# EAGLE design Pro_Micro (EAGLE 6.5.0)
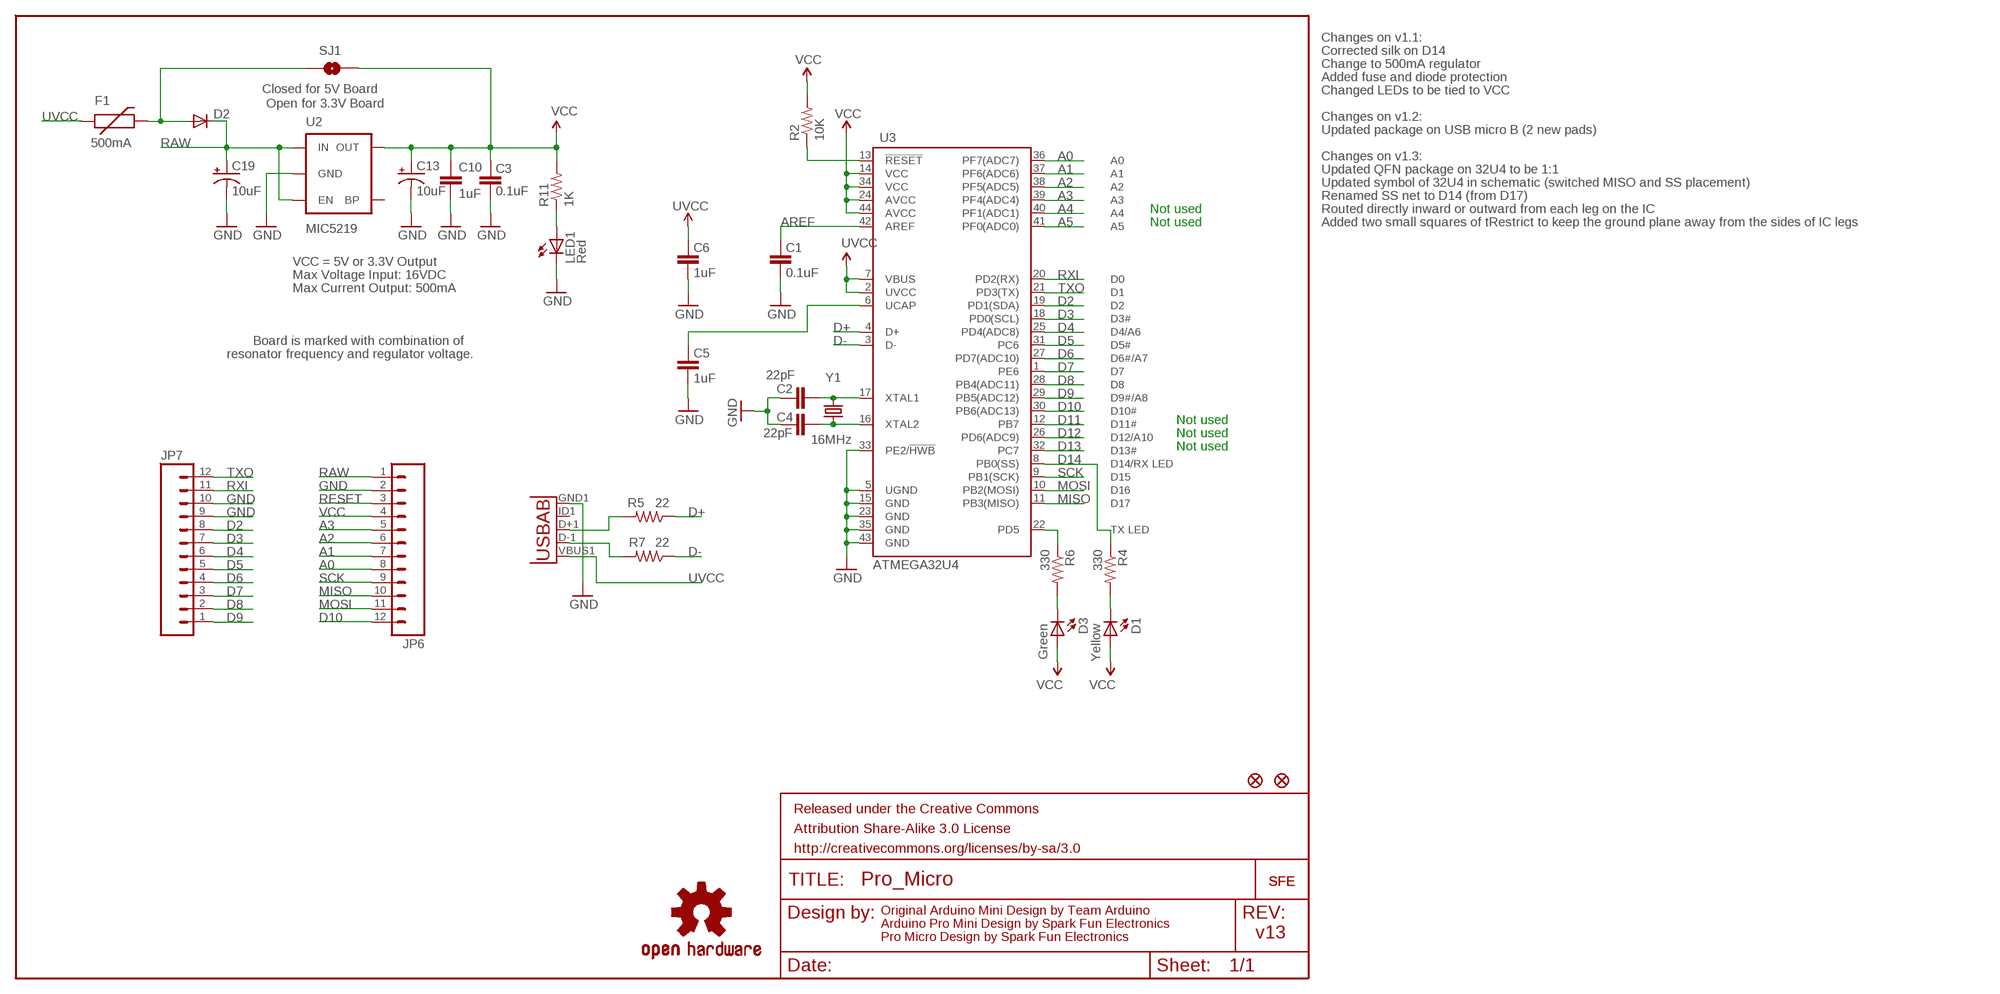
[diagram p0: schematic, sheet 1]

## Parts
C1  0.1uF  CAP0603-CAP  [0603-CAP]
C2  22pF  CAP0603-CAP  [0603-CAP]
C3  0.1uF  CAP0603-CAP  [0603-CAP]
C4  22pF  CAP0603-CAP  [0603-CAP]
C5  1uF  CAP0603-CAP  [0603-CAP]
C6  1uF  CAP0603-CAP  [0603-CAP]
C10  1uF  CAP0603-CAP  [0603-CAP]
C13  10uF  CAP_POL1206  [EIA3216]
C19  10uF  CAP_POL1206  [EIA3216]
D1  Yellow  LED0603  [LED-0603]
D2  DIODESOD  [SOD-323]
D3  Green  LED0603  [LED-0603]
F1  500mA  PTCSMD  [PTC-1206]
FRAME1  FRAME-LETTER  [CREATIVE_COMMONS]
JP1  FIDUCIALUFIDUCIAL  [MICRO-FIDUCIAL]
JP2  FIDUCIALUFIDUCIAL  [MICRO-FIDUCIAL]
JP6  M12PTH  [1X12]
JP7  M12PTH  [1X12]
LED1  Red  LED0603  [LED-0603]
R2  10K  RESISTOR0603-RES  [0603-RES]
R4  330  RESISTOR0603-RES  [0603-RES]
R5  22  RESISTOR0603-RES  [0603-RES]
R6  330  RESISTOR0603-RES  [0603-RES]
R7  22  RESISTOR0603-RES  [0603-RES]
R11  1K  RESISTOR0603-RES  [0603-RES]
SJ1  Closed for 5V Board  SOLDERJUMPERNO  [SJ_2S-NO]
U2  MIC5219  V_REG_LDOSMD  [SOT23-5]
U3  ATMEGA32U4  ATMEGA32U4OUTFAKES  [QFN-44-NOPAD_1:1-OUTFAKES]
U$1  LOGO-SFESK  [SFE-LOGO-FLAME]
U$3  OSHW-LOGOS  [OSHW-LOGO-S]
U$11  LOGO-SFENEW  [SFE-NEW-WEBLOGO]
X1  USB-ABIN&OUT  [USB-AB-MICRO-SMD-V03-IN&OUT]
Y1  16MHz  CRYSTAL5X3  [CRYSTAL-SMD-5X3]

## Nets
A0: JP6.8 U3.36(PF7(ADC7))
A1: JP6.7 U3.37(PF6(ADC6))
A2: JP6.6 U3.38(PF5(ADC5))
A3: JP6.5 U3.39(PF4(ADC4))
A4: U3.40(PF1(ADC1))
A5: U3.41(PF0(ADC0))
AREF: C1.2 U3.42(AREF)
D2: JP7.8 U3.19(PD1(SDA))
D3: JP7.7 U3.18(PD0(SCL))
D4: JP7.6 U3.25(PD4(ADC8))
D5: JP7.5 U3.31(PC6)
D6: JP7.4 U3.27(PD7(ADC10))
D7: JP7.3 U3.1(PE6)
D8: JP7.2 U3.28(PB4(ADC11))
D9: JP7.1 U3.29(PB5(ADC12))
D10: JP6.12 U3.30(PB6(ADC13))
D11: U3.12(PB7)
D12: U3.26(PD6(ADC9))
D13: U3.32(PC7)
D14: R4.1 U3.8(PB0(SS))
D+: R5.1 U3.4(D+)
D-: R7.1 U3.3(D-)
GND [vcc]: C1.1 C2.2 C3.1 C4.2 C5.1 C6.1 C10.2 C13.C(-) C19.C(-) JP6.2 JP7.9 JP7.10 LED1.C U2.2(GND) U3.5(UGND) U3.15(GND) U3.23(GND) U3.33(PE2/!HWB) U3.35(GND) U3.43(GND) X1.GND1(GND)
MISO: JP6.10 U3.11(PB3(MISO))
MOSI: JP6.11 U3.10(PB2(MOSI))
N$1: C4.1 U3.16(XTAL2) Y1.1
N$2: C2.1 U3.17(XTAL1) Y1.3
N$3: D2.2(A) F1.2 SJ1.1
N$4: C5.2 U3.6(UCAP)
N$5: D1.C R4.2
N$6: R7.2 X1.D-1(D-)
N$7: D3.C R6.2
N$8: R5.2 X1.D+1(D+)
N$38: LED1.A R11.1
RAW [vcc]: C19.A(+) D2.1(C) JP6.1 U2.1(IN) U2.3(EN)
RESET: JP6.3 R2.1 U3.13(!RESET)
RXI: JP7.11 U3.20(PD2(RX))
SCK: JP6.9 U3.9(PB1(SCK))
TXLED: R6.1 U3.22(PD5)
TXO: JP7.12 U3.21(PD3(TX))
UVCC: C6.2 F1.1 U3.2(UVCC) U3.7(VBUS) X1.VBUS1(VBUS)
VCC: C3.2 C10.1 C13.A(+) D1.A D3.A JP6.4 R2.2 R11.2 SJ1.2 U2.5(OUT) U3.14(VCC) U3.24(AVCC) U3.34(VCC) U3.44(AVCC)
Unconnected: U2.4(BP) X1.ID1(USBID)

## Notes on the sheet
- Changes on v1.1:
- Corrected silk on D14
- Change to 500mA regulator
- Added fuse and diode protection
- Changed LEDs to be tied to VCC
- Open for 3.3V Board
- Changes on v1.2:
- Updated package on USB micro B (2 new pads)
- Changes on v1.3:
- Updated QFN package on 32U4 to be 1:1
- Updated symbol of 32U4 in schematic (switched MISO and SS placement)
- Renamed SS net to D14 (from D17)
- Not used | Routed directly inward or outward from each leg on the IC
- Not used | Added two small squares of tRestrict to keep the ground plane away from the sides of IC legs
- VCC = 5V or 3.3V Output
- Max Voltage Input: 16VDC
- Max Current Output: 500mA
- Board is marked with combination of
- resonator frequency and regulator voltage.
- Not used
- Not used
- Not used
- Original Arduino Mini Design by Team Arduino
- Arduino Pro Mini Design by Spark Fun Electronics
- Pro Micro Design by Spark Fun Electronics | v13

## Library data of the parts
C1-C6 C10 = SparkFun:CAP: Capacitor
C13 C19 = SparkFun:CAP_POL: Capacitor Polarized
D1 D3 LED1 = SparkFun:LED: LEDs
D2 = SparkFun:DIODE: Diode
F1 = SparkFun:PTC: Resettable Fuse PTC
FRAME1 = SparkFun-Aesthetics:FRAME-LETTER: Schematic Frame
JP1 JP2 = SparkFun:FIDUCIAL: Fiducial Alignment Points
JP6 JP7 = SparkFun:M12: Header 12 Standard 12-pin 0.1" header. Use with straight break away headers (SKU : PRT-00116), right angle break away headers (PRT-00553), swiss pins (PRT-00743), machine pins (PRT-00117), and female headers (PRT-00115).
R2 R4-R7 R11 = SparkFun:RESISTOR: Resistor
SJ1 = SparkFun:SOLDERJUMPER: Solder Jumper
U2 = SparkFun:V_REG_LDO: Voltage Regulator LDO Standard 150mA LDO voltage regulator in SOT-23 layout. Micrel part MIC5205. BP (by-pass) pin is used to lower output noise with 470pF cap.
U3 = Testing:ATMEGA32U4: Atmel 44-pin 8-bit Microcontroller with 32KBytes of ISP Flash and USB Controller
U$1 U$11 = SparkFun:LOGO-SFE: Spark Fun Electronics PCB Logo
U$3 = SparkFun:OSHW-LOGO: Open Source Hardware Logo This logo indicates the piece of hardware it is found on incorporates a OSHW license and/or adheres to the definition of open source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
X1 = Testing:USB-AB: This is a USB AB connector that is compatible with USB OTG. i.e. this connector can serve as a host or device
Y1 = SparkFun:CRYSTAL: Crystals

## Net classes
0 default: width 0.203 mm

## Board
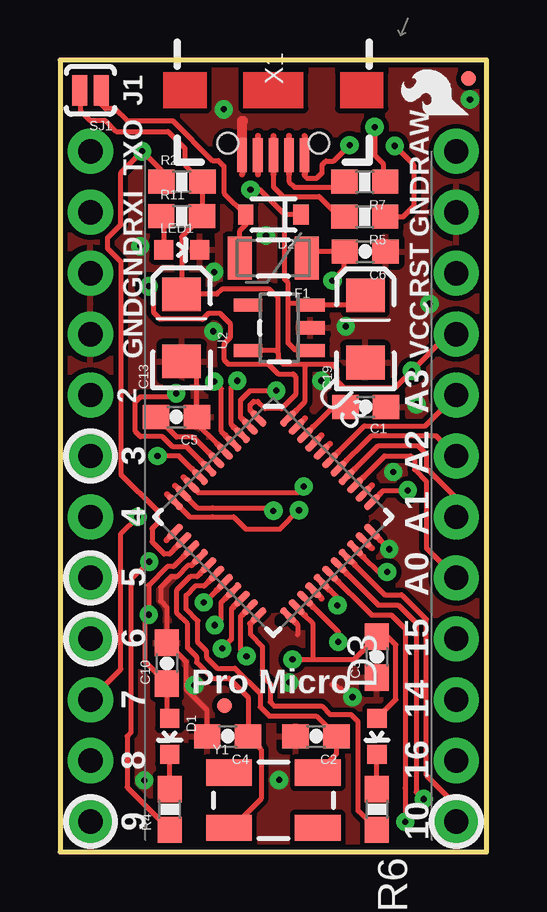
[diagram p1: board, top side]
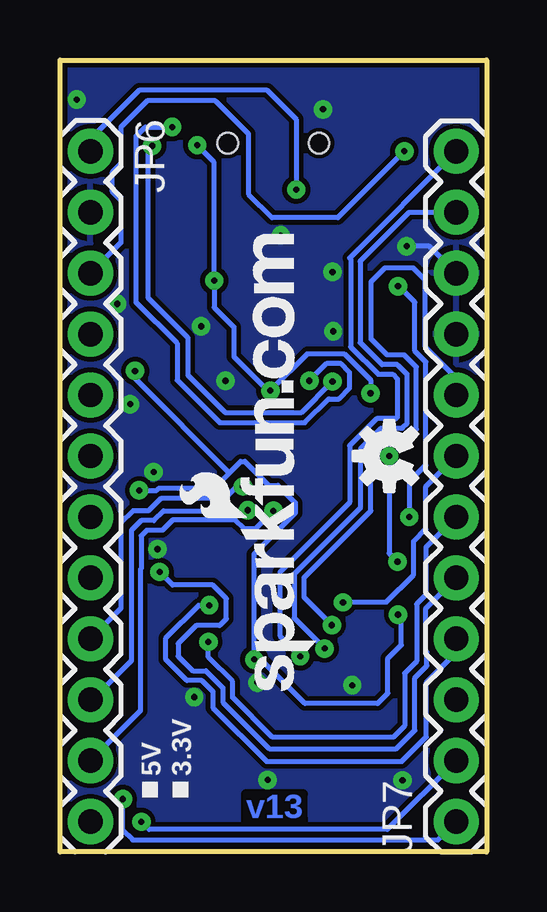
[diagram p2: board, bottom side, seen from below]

Size 17.78 x 33.02 mm. Coordinates in mm from the lower left corner, seen from the top.
Outline: 0,33.02 0,0 17.78,0 17.78,33.02 0,33.02
Copper layers (1*16): Top 0.035mm / dielectric 1.5mm / Bottom 0.035mm
Design rules "SparkFun *": minimum track width 8mil, minimum drill 15mil, track to track 7mil, track to pad 7mil, pad to pad 7mil, via to via 7mil, smd to smd 7mil, copper to edge 7mil, drill to drill 7mil, minimum pad ring 12mil, minimum via ring 10mil, stop-mask expansion 4mil, vias tented up to drill 20mil, thermal gap 10mil
tRestrict: area 9.1,9.6 to 9.3,9.7; area 13.1,13.6 to 13.1,13.7; area 5.5,10.3 to 12.6,17.6

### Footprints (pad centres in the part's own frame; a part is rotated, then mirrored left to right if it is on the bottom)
0603-CAP = smd 1.1 x 1: 1 -0.85,0; 2 0.85,0
EIA3216 = smd 1.4 x 1.6: A 1.4,0; C -1.4,0
LED-0603 = smd 0.8 x 0.8: A 0,-0.75; C 0,0.75
SOD-323 = smd 0.63 x 0.83: 1 -1.15,0; 2 1.15,0
PTC-1206 = smd 1 x 1.8: 1 -1.4,0; 2 1.4,0
MICRO-FIDUCIAL = smd 0.635 x 0.635: 1 0,0
1X12 = drill 1.016 pad 1.88: 1 0,0; 2 2.54,0; 3 5.08,0; 4 7.62,0; 5 10.16,0; 6 12.7,0; 7 15.24,0; 8 17.78,0; 9 20.32,0; 10 22.86,0; 11 25.4,0; 12 27.94,0
0603-RES = smd 1.1 x 1: 1 -0.85,0; 2 0.85,0
SJ_2S-NO = smd 0.635 x 1.27: 1 -0.45,0; 2 0.45,0
SOT23-5 = smd 0.55 x 1.2: 1 -0.95,-1.3; 2 0,-1.3; 3 0.95,-1.3; 4 0.95,1.3; 5 -0.95,1.3
QFN-44-NOPAD_1:1-OUTFAKES = smd 0.8 x 0.3: 1 -3.337,2.465; 2 -3.337,1.972; 3 -3.337,1.479; 4 -3.337,0.986; 5 -3.337,0.493; 6 -3.337,0; 7 -3.337,-0.493; 8 -3.337,-0.986; 9 -3.337,-1.479; 10 -3.337,-1.972; 11 -3.337,-2.465; 23 3.337,-2.465; 24 3.337,-1.972; 25 3.337,-1.479; 26 3.337,-0.986; 27 3.337,-0.493; 28 3.337,0; 29 3.337,0.493; 30 3.337,0.986; 31 3.337,1.479; 32 3.337,1.972; 33 3.337,2.465 | smd 0.3 x 0.8: 12 -2.465,-3.337; 13 -1.972,-3.337; 14 -1.479,-3.337; 15 -0.986,-3.337; 16 -0.493,-3.337; 17 0,-3.337; 18 0.493,-3.337; 19 0.986,-3.337; 20 1.479,-3.337; 21 1.972,-3.337; 22 2.465,-3.337; 34 2.465,3.337; 35 1.972,3.337; 36 1.479,3.337; 37 0.986,3.337; 38 0.493,3.337; 39 0,3.337; 40 -0.493,3.337; 41 -0.986,3.337; 42 -1.479,3.337; 43 -1.972,3.337; 44 -2.465,3.337
USB-AB-MICRO-SMD-V03-IN&OUT = smd 1.4 x 0.4: D+1 2.7,0; D-1 2.7,0.65; GND1 2.7,-1.3; ID1 2.7,-0.65; VBUS1 2.7,1.3 | hole 0.85: 2.2,1.9; 2.2,-1.9
CRYSTAL-SMD-5X3 = smd 1.9 x 1.1: 1 -1.85,-1.15; 2 1.85,-1.15; 3 1.85,1.15; 4 -1.85,1.15

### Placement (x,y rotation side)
C1  12.74,18.56 180 top
C2  10.67,4.83 180 top
C3  13.21,8.13 90 top
C4  6.99,4.83 180 top
C5  4.85,18.14 180 top
C6  12.71,25.03 180 top
C10  4.46,7.87 90 top
C13  5.07,21.85 90 top
C19  12.72,21.8 90 top
D1  4.57,4.83 180 top
D2  8.89,26.57 180 top
D3  13.21,4.83 180 top
F1  8.89,24.77 180 top
FRAME1  not placed on the board
JP1  6.86,6.1 0 top
JP2  17.02,32.26 0 top
JP6  16.51,29.21 270 bottom
JP7  1.27,1.27 90 bottom
LED1  5.07,25.11 270 top
R2  5.08,27.94 0 top
R4  4.57,1.78 90 top
R5  12.7,26.49 180 top
R6  13.21,1.78 90 top
R7  12.7,27.94 180 top
R11  5.07,26.5 0 top
SJ1  1.27,31.75 180 top
U2  9.14,21.85 90 top
U3  8.89,13.97 315 top
U$1  17.02,30.73 90 top
U$3  4.06,16.51 90 bottom
U$11  7.11,6.73 90 bottom
X1  8.89,31.75 270 top
Y1  8.89,2.16 0 top

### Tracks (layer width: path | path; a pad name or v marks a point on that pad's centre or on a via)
A0
  Top 0.203: U3.36 13.53,16.52 14.61,16.52 14.78,16.35 14.78,15.94 15.27,15.45 15.27,12.67 JP6.8
A1
  Top 0.203: U3.37 13.26,16.95 14.91,16.95 15.27,16.59 15.27,16.01 16.51,14.77 JP6.7
A2
  Top 0.203: U3.38 12.98,17.36 15.66,17.36 JP6.6
A3
  Top 0.203: 12.68,17.77 12.69,17.77 | 11.6,16.68 12.69,17.77 | 12.69,17.77 15.22,17.77 JP6.5
AREF
  Top 0.203: 10.55,17.72 11.39,18.56 C1.2
D2  (via drill 0.25)
  Top 0.203: 6.88,10.56 6.71,10.39 6.71,9.72 v6.45,9.46
  Bottom 0.203: v6.45,9.46 7.62,10.63 7.62,11.43 4.83,14.22 4.83,16.69 4.23,17.29 3.28,17.29 2.93,17.63 2.93,20.22 3.44,20.73 4.15,20.73 4.82,21.4 4.82,23.77 4.83,23.77 4.25,24.35 3.06,24.35 2.55,23.85 2.55,21.05 1.27,19.76 JP7.8
D3  (via drill 0.25)
  Top 0.203: 6.53,10.91 6.02,10.41 v5.99,10.41
  Bottom 0.203: JP7.7 2.54,15.24 2.54,13.46 3.05,12.95 3.05,11.56 4.2,10.41 v5.99,10.41
D4  (via drill 0.25)
  Top 0.203: 10.55,10.22 11.6,9.17 v11.6,8.76
  Bottom 0.203: JP7.6 2.54,12.7 2.54,10.72 2.92,10.34 2.92,7.95 3.42,7.45 3.42,5.26 3.89,4.79 8.93,4.79 10.58,6.45 10.58,7.1 11.6,8.12 v11.6,8.76
D5  (via drill 0.25)
  Top 0.203: 12.64,12.31 13.28,11.68 v13.63,11.68
  Bottom 0.203: JP7.5 2.54,10.16 2.54,8.38 2.5,8.34 2.5,7.76 3,7.27 3,5.07 3.76,4.3 9.05,4.3 11,6.25 11,6.86 11.01,6.86 11.71,7.55 12.25,7.55 12.86,8.16 12.86,8.69 12.11,9.44 11.13,9.44 10.85,9.73 10.85,10.57 11.41,11.13 13.09,11.13 v13.63,11.68
D6  (via drill 0.25)
  Top 0.203: v11.56,10.29 11.56,10.6 v11.56,10.29 | U3.27 11.56,10.61 v11.56,10.29
  Bottom 0.203: v11.56,10.29 12.01,10.29 13.37,8.92 13.37,8.03 12.49,7.15 11.87,7.15 11.41,6.69 11.41,6.02 9.17,3.78 3.53,3.78 2.51,4.8 2.51,7.07 1.27,8.31 JP7.4
D7  (via drill 0.25)
  Top 0.203: JP7.3 2.54,7.62 2.54,13.28 v3.23,13.97 | v3.7,23.59 3.7,23.54 3.91,23.32 3.91,22.48 4.17,22.22 5.95,22.22 6.19,22.46 6.66,22.46 7.09,22.04 7.09,21.44 6.84,21.2 6.84,20.51 7.03,20.33 8.71,20.33 8.71,20.31 9.1,19.93 9.72,19.93 9.82,19.83 9.82,19.07 9.24,18.49 8.54,18.49 8.24,18.79 8.07,18.79 7.92,18.64 7.92,18.43 U3.1 7.93,18.42
  Bottom 0.203: v3.7,23.59 3.67,23.59 3,22.92 3,20.89 2.54,20.43 2.54,16.13 3.23,15.44 v3.23,13.97
D8  (via drill 0.25)
  Top 0.203: U3.28 12.98,9.88 13.8,9.88 14.38,9.31 14.38,2.67 14.39,2.65 v14.39,1.26
  Bottom 0.203: JP7.2 4.14,0.94 14.07,0.94 v14.39,1.26
D9  (via drill 0.25)
  Top 0.203: 11.95,11.61 13.26,10.3 14.08,10.3 14.83,9.55 14.83,2.49 15.12,2.21 v15.16,2.21
  Bottom 0.203: JP7.1 2.03,0.51 14.76,0.51 15.16,0.91 v15.16,2.21
D10
  Top 0.203: JP6.12 16.51,1.96 15.27,3.2 15.27,9.7 14.24,10.73 13.53,10.73 U3.30
D14  (via drill 0.25)
  Top 0.203: R4.1 2.79,2.71 2.79,4.83 2.95,4.98 2.95,11.34 v3.72,12.1 | 5.5,15.97 4.96,16.51 v4.06,16.51
  Bottom 0.203: v4.06,16.51 4.06,12.45 v3.72,12.1
D+  (via drill 0.25)
  Top 0.203: v13.95,29.44 14.73,28.65 14.73,26.92 14.29,26.49 R5.1 | U3.4 6.72,17.53 6.72,19.32 v6.43,19.61
  Bottom 0.203: v13.95,29.44 14.1,29.29 14.1,23.09 12.45,21.44 12.45,19.88 10.91,18.34 10.91,18.32 7.72,18.32 v6.43,19.61
D-  (via drill 0.25)
  Top 0.203: 13.55,28.26 R7.1 13.46,28.03 13.46,28.7 13.11,29.06 v13.11,30.23 | v7.39,19.65 7.14,19.39 7.14,17.81 7.24,17.71
  Bottom 0.203: v13.11,30.23 14.22,30.23 14.61,29.84 14.61,22.91 12.9,21.21 12.9,19.67 11.12,17.9 7.57,17.9 6.58,18.89 6.18,18.89 6.17,18.88 5.72,19.34 5.72,20 6.07,20.36 6.68,20.36 v7.39,19.65
GND  (via drill 0.25)
  Top 0.203: v13.71,12.62 v13.72,12.62 | U3.33 13.65,12.7 13.97,12.7 | C3.1 13.21,7.47 | 5.49,11.96 5.36,11.96 4.9,11.5 4.66,11.5 4.2,11.03 4.2,10.46 4.46,10.2 C10.2 4.63,8.55 4.64,8.55 5.26,7.92 5.26,6.78 6.13,5.91 C4.2 | 9.86,9.52 9.91,9.47 9.91,9.07 | 11.34,6.98 arc-21 v12.19,6.46 | 5.38,20.45 C13.C 5.7,19.82 C5.1 5.7,17.85 6.54,17.02
  Top 0.406: X1.GND1 7.59,30.48 7.62,30.48
  Bottom 0.203: JP7.10 2.39,25.25 v3.34,25.25
  other vias: 9.13,3 14.86,18.67 11.9,21.92 13.88,15.84 10.88,19.65 6.39,21.71 17.08,31.37 8.58,25.7 15.4,22.85 6.82,30.96 3.51,2.99 5.6,6.95 6.43,24.18 9.56,7.06
  pour Top (isolate 0.203): 0,33.02 17.78,33.02 17.78,0 0,0
  pour Bottom (isolate 0.203): 0,33.02 17.78,33.02 17.78,0 0,0
MISO  (via drill 0.25)
  Top 0.203: v9.96,14.25 9.17,13.46 7.75,13.46 7.24,13.97 6.35,13.97 5.42,13.97 5.4,13.97 U3.11
  Bottom 0.203: JP6.10 16.43,6.35 14.81,7.98 14.81,13.41 14.4,13.82 13.87,13.82 13.46,14.22 9.98,14.22 v9.96,14.25
MOSI  (via drill 0.25)
  Top 0.203: v8.89,14.22 8.76,14.35 6.35,14.35 5.74,14.35 5.72,14.35 U3.10
  Bottom 0.203: JP6.11 14.43,5.89 14.43,11.79 14.4,11.81 14.4,13.18 14.17,13.41 13.51,13.41 13.08,13.84 10.49,13.84 10.11,13.46 9.65,13.46 v8.89,14.22
N$1
  Top 0.203: Y1.1 7.17,1.01 8.38,2.22 8.38,4.28 C4.1 7.83,6.45 7.05,7.24 6.35,7.24 5.69,7.9 5.69,8.14 5.32,8.51 5.32,9.51 4.85,9.98 4.85,10.9 | 5.83,11.61 5.71,11.49 5.44,11.49 4.85,10.9 | 4.85,10.9
N$2
  Top 0.203: Y1.3 11.52,4.09 C2.1 10.68,5.67 8.71,5.67 8.34,6.04 8.34,6.61 7.29,7.67 6.55,7.67 6.1,8.12 6.1,8.37 5.74,8.73 5.74,9.64 5.25,10.13 5.25,10.71 5.63,11.09 6,11.09 6.18,11.26
N$3
  Top 0.203: F1.2 7.49,25.91 7.74,26.16 D2.2 6.83,27.48 6.83,28.6 6.6,28.83 6.35,28.83 4.7,30.48 2.79,30.48 2.29,30.99 1.91,30.99 1.68,31.21 SJ1.1
N$4
  Top 0.203: C5.2 4.03,18.14 4.86,17.3 5.56,17.3 U3.6
N$5
  Top 0.203: R4.2 D1.C
N$6
  Top 0.203: X1.D-1 9.54,27.95 9.78,27.71 11.65,27.71 11.85,27.91 R7.2
N$7
  Top 0.203: R6.2 D3.C
N$8
  Top 0.203: X1.D+1 8.89,27.74 9.3,27.33 10.79,27.33 11.64,26.49 R5.2
N$38
  Top 0.203: R11.1 4.32,26.4 LED1.A
RAW  (via drill 0.25)
  Top 0.203: 9.51,22.86 9.51,21.21 9.78,20.94 10.4,20.94 U2.1 | D2.1 9.37,26.57 | 9.37,26.57 8.33,27.61 v7.94,27.61 | C19.A 12.32,22.8 U2.3 10.38,22.86 9.51,22.86 | 9.51,22.86 9.51,23.73 9.36,23.88 9.36,26.56 9.37,26.57
  Bottom 0.203: JP6.1 16.51,29.72 14.48,31.75 9.14,31.75 7.94,30.54 v7.94,27.61
RESET  (via drill 0.25)
  Top 0.203: 4.79,12.66 4.71,12.58 4.71,12.57 4.56,12.42 4.34,12.42 3.83,12.93 3.83,13.49 4.06,13.72 4.06,14.22 2.54,15.75 2.54,24.61 1.98,25.17 1.98,25.59 2.54,26.15 2.54,28.32 v3.43,29.21 4.23,28.41 R2.1
  Bottom 0.203: JP6.3 15.24,25.4 15.24,27.18 15.62,27.56 15.62,28.32 15.24,28.7 15.24,30.23 14.15,31.32 11.3,31.32 9.93,29.95 9.93,27.43 8.94,26.44 6.2,26.44 v3.43,29.21
RXI  (via drill 0.25)
  Top 0.203: 7.23,10.22 7.14,10.13 7.14,8.87 v6.75,8.48
  Bottom 0.203: JP7.11 3.23,26.67 5.27,24.63 5.27,21.23 4.36,20.32 3.72,20.32 3.72,20.31 3.32,19.91 3.32,17.87 3.52,17.67 | v6.75,8.48 8.03,9.76 8.03,11.6 5.26,14.37 5.26,16.82 4.4,17.67 3.52,17.67 | 3.52,17.67 3.51,17.67
SCK  (via drill 0.25)
  Top 0.203: v10.16,15.24 9.91,14.99 6.35,14.99 5.78,14.99 | 5.75,14.99 5.78,14.99 | U3.9 5.78,14.99
  Bottom 0.203: JP6.9 15.24,10.16 15.24,13.72 14.73,14.22 14.1,14.22 13.59,14.73 10.92,14.73 10.41,15.24 v10.16,15.24
TXLED
  Top 0.203: 7.92,9.52 7.93,9.53 7.94,9.53 7.94,9.05 8.44,8.55 8.44,7.34 8.75,7.03 8.75,6.25 8.91,6.09 10.9,6.09 11.27,5.72 12.13,5.72 12.42,5.44 12.42,1.72 R6.1
TXO  (via drill 0.25)
  Top 0.203: 7.58,9.87 7.54,9.83 7.52,9.83 7.52,8.41 v7.77,8.16
  Bottom 0.203: JP7.12 5.71,24.77 5.67,24.72 5.67,21.05 4.53,19.92 3.92,19.92 3.72,19.72 3.72,18.13 3.79,18.06 4.59,18.06 5.71,16.94 5.71,14.57 8.62,11.66 8.62,9.01 v7.77,8.16
UVCC  (via drill 0.25)
  Top 0.203: 10.42,24.89 F1.1 10.56,25.03 C6.2 11.85,24.32 v11.35,23.82 | v12.06,29.46 11.4,28.8 11.07,28.8 10.92,28.65 10.92,28.32 10.69,28.09 10.29,28.09 10.19,28.19 X1.VBUS1 | v9.01,19.23 7.92,19.23 7.52,18.84 7.52,18.11 7.54,18.11 7.59,18.06 | v4.84,19.12 4.7,18.99 3.35,18.99 3.14,18.77 3.14,17.53 3.35,17.32 4.26,17.32 4.68,16.91 5.29,16.91 5.29,16.87 U3.7
  Bottom 0.203: 11.43,23.9 v11.35,23.82 | v11.35,23.82 11.35,28.75 v12.06,29.46 | v11.35,23.82 11.35,22.7 10.54,21.89 10.54,20.65 9.12,19.23 v9.01,19.23 7.46,20.78 5.94,20.78 4.84,19.68 v4.84,19.12
VCC  (via drill 0.25)
  Top 0.203: SJ1.2 0.86,30.89 1.27,30.48 1.91,30.48 2.35,30.04 4.51,30.04 5.21,29.34 5.21,28.66 R2.2 5.92,27.93 R11.2 5.07,25.65 C13.A | C3.2 13.65,8.98 13.99,8.64 13.99,6.36 D3.A | 4.28,7.02 C10.1 | 4.52,5.63 D1.A 4.46,5.69 C10.1 | 5.14,12.31 4.73,11.9 4.47,11.9 3.7,11.12 v3.7,9.9 3.56,9.76 3.56,7.93 C10.1 | 12.97,8.98 C3.2 | 10.2,9.87 10.53,9.54 10.53,8.08 arc90 10.58,8.02 | U3.34 13.47,15.06 14.47,15.06 v14.49,15.08 | C13.A 5.45,23.25 | 9.09,20.8 9.09,23.1 8.73,23.46 6.75,23.46 6.54,23.25 C13.A | 9.09,20.8 arc90 8.98,20.9 U2.5 | 10.28,20.33 11.35,20.33 11.55,20.12 11.55,19.64 11.83,19.36 13.96,19.36 v14.65,20.06 16.18,21.59 JP6.4 16.37,21.59 | 10.28,20.33 9.32,20.33 9.09,20.56 9.09,20.8 | 10.28,20.33 10.22,20.26 10.22,18.78 9.86,18.42 | v9.69,8.02 10.58,8.02 | 10.58,8.02 12.25,8.02 C3.2
  Bottom 0.203: v3.7,9.9 3.56,9.76 3.56,8.63 4.12,8.07 4.12,6.62 4.54,6.19 7.57,6.19 9.41,8.02 v9.69,8.02 arc90 9.7,8.03 9.7,12.41 7.97,14.14 7.97,14.55 8.71,15.29 9.08,15.29 10.08,16.28 10.26,16.28 10.73,15.81 | v14.49,15.08 13.75,15.08 13.66,15.17 11.37,15.17 10.73,15.81 | v14.65,20.06 14.65,19.73 10.73,15.81

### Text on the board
Bottom: v13
tPlace: J1 | TXO | RAW | RXI | GND | GND | RST | GND | VCC | 2 | A3 | 3 | A2 | 4 | A1 | 5 | A0 | 6 | 15 | Pro | Micro | 7 | 14 | 8 | 16 | 9 | 10
bPlace: 3.3V | 5V
tValues: Valid combinations: | 3.3V Reg / 8MHz | 5V Reg / 16MHz | Mark back accordingly
tDocu: N. Seidle, revised by P. Lewis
